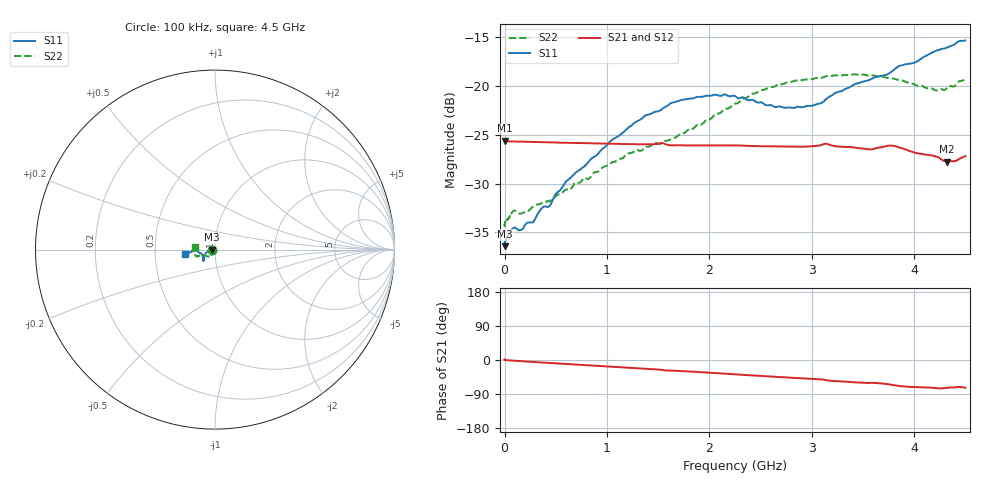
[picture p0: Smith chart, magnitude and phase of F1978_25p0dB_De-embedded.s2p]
! Integrated Device Technology
! Corporate Headquarters
! 6024 Silver Creek Valley Road
! San Jose, CA 95138  USA
! Phone:  1-408-284-8200
! Toll Free:  1-800-223-1366
! Webpage:  http://www.idt.com/
! Timing and RF Division
! 515 Groton Road, Suite 102
! Westford, MA 01886-6024
! Device:  F1978
! Description: 6-bit, 75 ohm, 0.5 dB Digital Step Attenuator
! Frequency:  5.0 MHz -  3.00 GHz
! Package:  4x4 mm QFN Plastic Package: 20 pin
! Ports:  2 RF, 11 DC
!  Pin  1  = D5 (16 dB)
!  Pin  2  = RF1  =  Port 1
!  Pin  3  = Serial Data In (DATA)
!  Pin  4  = Serial Clock (CLK)
!  Pin  5  = Serial Latch Enable (LE)
!  Pin  6  = VDD
!  Pin  7  = NC
!  Pin  8  = NC
!  Pin  9  = NC
!  Pin 10  = GND
!  Pin 11  = GND
!  Pin 12  = NC
!  Pin 13  = VMODE
!  Pin 14  = RF2  =  Port 2
!  Pin 15  = D4 (8 dB)
!  Pin 16  = D3 (4 dB)
!  Pin 17  = D2 (2 dB)
!  Pin 18  = NC
!  Pin 19  = D1 (1 dB)
!  Pin 20  = D0 (0.5 dB)
! State:  50
! Atten State:  25.0 dB
! Voltage:  +3.30 Volts
! Current:  0.593 mA
! Data:  The device was measured on a F1975 evaluation board which has
!  individual transmission lines to the RF pins.  Data was collected
!  using a calibrated network analyzer.  The evaluation board was
!  de-embedded using Automatic Fixture Removal (AFR).
!  The reference plane is the edge of the package pin.
! Misc:
!  Action Tracker AT0416
! Date Measured:  2018-02-08
! Date:  2018-03-26  MJV
! Note:
!  Integrated Device Technology supplies this data as a sample of measured
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# GHz S dB R 75
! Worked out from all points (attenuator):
!   291 points, 100 kHz to 4.5 GHz, reference 75 ohm
!   highest |S21| = -25.60 dB at 300 kHz (marker M1); lowest = -27.7 dB at 4.32 GHz (marker M2)
!   lowest |S11| = -36.4 dB at 100 kHz (marker M3), VSWR 1.03, Z = 72.8 + j0.0186 ohm
!   |S11| at or under -10 dB: start of sweep to end of sweep
!   |S22| runs from -34.4 to -18.8 dB; largest |S21 - S12| = 0.00017
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0.0001  -36.43 179.5  -25.61 1.2  -25.59 1.3  -34.30 -178.8
0.0003  -36.39 -179.5  -25.60 1.1  -25.61 1.1  -34.30 -178.8
0.014  -35.69 -178.0  -25.67 -0.4  -25.66 -0.4  -33.80 -176.0
0.08  -34.60 -176.0  -25.68 -1.6  -25.68 -1.6  -32.85 -168.6
0.16  -34.77 -177.2  -25.71 -3.1  -25.70 -3.1  -33.10 -158.6
0.28  -33.96 180.0  -25.73 -5.2  -25.73 -5.2  -32.36 -149.5
0.36  -32.57 179.9  -25.76 -6.6  -25.76 -6.6  -32.01 -141.9
0.44  -32.32 -179.2  -25.77 -7.9  -25.77 -7.9  -31.85 -136.0
0.6  -29.79 -175.7  -25.82 -10.6  -25.82 -10.6  -30.60 -130.2
0.76  -28.38 -168.8  -25.85 -13.3  -25.85 -13.3  -29.63 -126.7
1.28  -23.68 -152.5  -25.96 -21.7  -25.96 -21.7  -26.60 -123.4
1.52  -22.50 -145.3  -25.86 -25.5  -25.87 -25.5  -25.94 -130.0
1.64  -21.69 -142.5  -26.08 -28.0  -26.08 -28.0  -25.35 -134.0
1.88  -21.11 -138.5  -26.09 -31.5  -26.09 -31.5  -23.99 -146.1
2.26  -21.09 -137.1  -26.10 -37.9  -26.09 -37.9  -21.78 -157.1
2.64  -22.15 -147.5  -26.18 -44.2  -26.18 -44.2  -20.02 -158.9
3.02  -21.96 -164.1  -26.15 -50.0  -26.15 -50.0  -19.24 -159.8
3.42  -19.81 -175.6  -26.32 -58.9  -26.32 -58.9  -18.78 -164.3
3.76  -18.66 -175.9  -26.10 -64.5  -26.10 -64.5  -19.17 -169.9
4.2  -16.43 -172.7  -27.19 -73.9  -27.18 -73.9  -20.43 178.6
4.32  -16.05 -172.1  -27.75 -73.5  -27.74 -73.5  -20.22 176.2
4.5  -15.31 -171.9  -27.19 -73.1  -27.19 -73.1  -19.18 173.6
